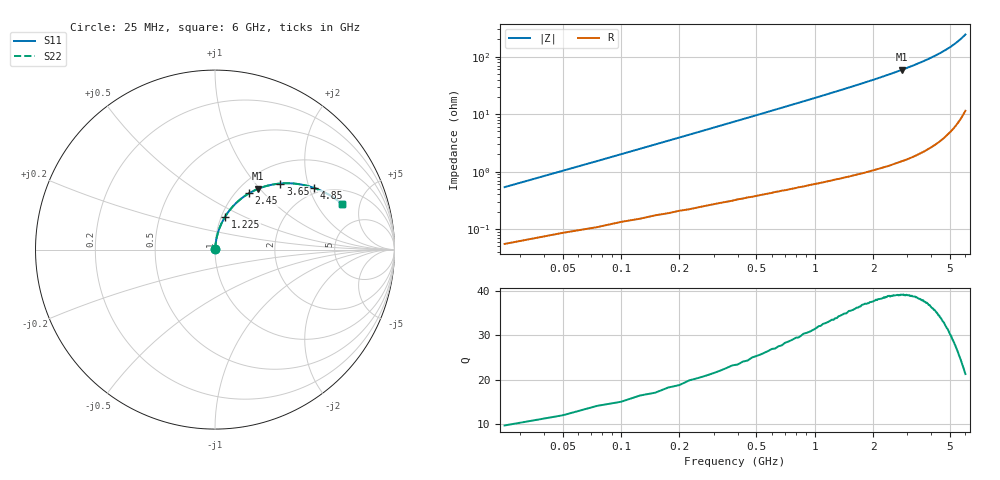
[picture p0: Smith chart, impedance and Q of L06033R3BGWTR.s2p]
!	AVX Thin Film Operation
!	Date:	March	2003
!	Description: Accu-L® Series Thin Film SMD RF Inductors
!	Part Number: L06033R3BGWTR
!	25MHz-6GHz
!	Serial	Measurements
#	mhz	S	db	R	50
!	S11	S11	S21	S21	S12	S12	S22	S22
!	dB	Phase	dB	Phase	dB	Phase	dB	Phase
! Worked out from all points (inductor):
!   240 points, 25 MHz to 6 GHz, reference 50 ohm
!   read as 1/Y11, port 2 shorted: L = 3.22 nH near 50 MHz
!   highest Q = 39.1 at 2.825 GHz (marker M1), where L = 3.34 nH
!   S11 on the Smith chart (normalised r, x): 25 MHz: 1.00, +0.01; 1.225 GHz: 1.04, +0.40; 2.45 GHz: 1.15, +0.83; 3.65 GHz: 1.36, +1.37; 4.85 GHz: 1.80, +2.14; 6 GHz: 2.90, +3.41
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25  -46.66 83.0  -0.01 -0.3  -0.01 -0.3  -46.66 83.0
50  -41.01 83.9  -0.01 -0.7  -0.01 -0.7  -41.01 83.9
75  -37.67 84.2  -0.01 -1.0  -0.01 -1.0  -37.67 84.2
100  -35.29 84.3  -0.01 -1.3  -0.01 -1.3  -35.29 84.3
125  -33.44 84.3  -0.01 -1.6  -0.01 -1.6  -33.44 84.3
175  -30.64 84.1  -0.02 -2.3  -0.02 -2.3  -30.64 84.1
275  -26.86 83.3  -0.03 -3.5  -0.03 -3.5  -26.86 83.3
400  -23.72 82.1  -0.05 -5.0  -0.05 -5.0  -23.72 82.1
575  -20.68 80.3  -0.07 -7.2  -0.07 -7.2  -20.68 80.3
775  -18.17 78.1  -0.11 -9.6  -0.11 -9.6  -18.17 78.1
1025  -15.84 75.2  -0.17 -12.7  -0.17 -12.7  -15.84 75.2
1225  -14.35 72.9  -0.22 -15.1  -0.22 -15.1  -14.35 72.9
1600  -12.15 68.6  -0.34 -19.5  -0.34 -19.5  -12.15 68.6
2025  -10.24 63.7  -0.52 -24.6  -0.52 -24.6  -10.24 63.7
2450  -8.72 58.8  -0.72 -29.5  -0.72 -29.5  -8.72 58.8
2825  -7.62 54.6  -0.93 -33.9  -0.93 -33.9  -7.62 54.6
3025  -7.10 52.3  -1.06 -36.1  -1.06 -36.1  -7.10 52.3
3650  -5.71 45.3  -1.50 -43.2  -1.50 -43.2  -5.71 45.3
4025  -5.02 41.1  -1.80 -47.4  -1.80 -47.4  -5.02 41.1
4850  -3.76 32.1  -2.57 -56.4  -2.57 -56.4  -3.76 32.1
5025  -3.54 30.2  -2.75 -58.3  -2.75 -58.3  -3.54 30.2
6000  -2.46 19.7  -3.93 -68.7  -3.93 -68.7  -2.46 19.7
